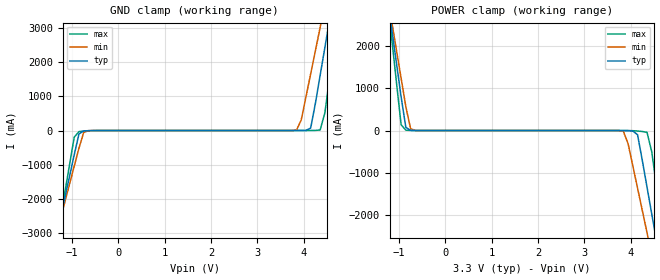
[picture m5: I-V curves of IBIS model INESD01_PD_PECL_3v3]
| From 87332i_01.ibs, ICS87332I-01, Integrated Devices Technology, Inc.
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[Model] INESD01_PD_PECL_3v3
Model_type  Input
Polarity   Non-Inverting
Vinl = 0.8V
Vinh = 2.0V
|   typ   min   max
C_comp   2pF   1.5pF   2.5pF
|   typ   min   max
[Voltage range]  3.3V   3.15V   3.45V
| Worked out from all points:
|   GND clamp passes 1 mA (typ) near -0.55 V on its own axis
|   POWER clamp passes 1 mA (typ) near -0.66 V on its own axis
[GND_clamp]
|Voltage   I(typ)   I(min)   I(max)
-2.586V   -10.86A    -9.487A    -13.15A
-1.361V   -3.24A     -3.145A    -3.432A
-1.259V   -2.606A    -2.617A    -2.622A
-952.6mV  -705.3mA   -1.038A    -192.4mA
-850.5mV  -99.9mA    -513.5mA   -31.23mA
-646.4mV  -3.788mA   -3.549mA   -8.297mA
3.844V    129.1uA    13.13mA    71.12uA
4.151V    73.33mA    1.652A     864.7uA
4.355V    1.607A     3.003A     15.44mA
4.559V    3.233A     4.356A     1.553A
4.763V    4.861A     5.711A     3.635A
5.375V    9.757A     9.783A     9.893A
[POWER_clamp]
|Voltage   I(typ)   I(min)   I(max)
-2.177V   10.57A     9.364A     12.62A
-1.157V   2.42A      2.586A     2.194A
-952.6mV  795.8mA    1.237A     137.8mA
-850.5mV  73.33mA    563.2mA    8.145mA
-646.4mV  535.8uA    2.004mA    431.2uA
3.844V    -826.3uA   -18.14mA   -47.07uA
4.151V    -99.9mA    -1.362A    -11.82mA
4.355V    -1.338A    -2.415A    -41.71mA
4.559V    -2.606A    -3.47A     -1.312A
4.661V    -3.24A     -3.998A    -2.123A
4.763V    -3.875A    -4.526A    -2.933A
5.579V    -8.954A    -8.756A    -9.414A
